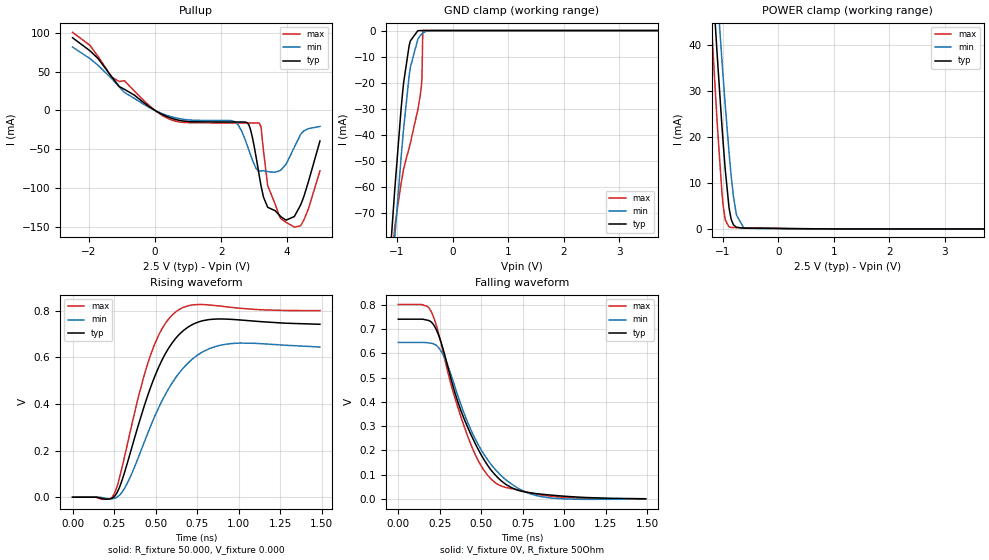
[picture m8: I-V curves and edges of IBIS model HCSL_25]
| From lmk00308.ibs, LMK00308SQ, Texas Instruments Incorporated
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|   Model HCSL_25
[Model]   HCSL_25
Model_type   Open_source
Polarity   Non-Inverting
Rref =   50.0000
Vref =   1.25
Vmeas =   1.25
|   typ   min   max
C_comp   1.5032pF   1.4574pF   1.5495pF
|Output in low   Nom   Weak   Strong
|C_Comp   1.5032pF   1.4574pF   1.5495pF
|Output in High   Nom   Strong   Weak
|C_Comp   1.0889pF   1.0724pF   1.10585pF
[Voltage Range]   2.5   2.375   2.625
[Temperature Range]   45   125   -40
[Pullup Reference]   2.5   2.375   2.625
[Pulldown Reference]   0   0   0
[Power Clamp Reference]   2.5   2.375   2.625
[GND Clamp Reference]   0   -0   0
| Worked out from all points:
|   slope of the pullup table from 0 to 0.375 V, typ, clamps not added: 46.2 ohm
|   GND clamp passes 1 mA (typ) near -0.66 V on its own axis
|   POWER clamp passes 1 mA (typ) near -0.81 V on its own axis
|   falling waveform, V_fixture 0V, R_fixture 50Ohm: 20-80 % time 248ps typ, 260ps min, 222ps max; typ from 0.74 V to 0.001 V
|   rising waveform, R_fixture 50.000, V_fixture 0.000: 20-80 % time 212ps typ, 251ps min, 177ps max; typ from 0 V to 0.742 V
[GND Clamp]
|   Voltage   I(typ)   I(min)   I(max)
-2.5V     -680.7mA   -652.3mA   -694.7mA
-1.135V   -89.97mA   -107.4mA   -101.7mA
-1.045V   -62.74mA   -81.12mA   -76.76mA
-1.038V   -60.54mA   -78.99mA   -75.08mA
-925mV    -30mA      -48.72mA   -58.7mA
-880mV    -20.04mA   -37.72mA   -53.1mA
-760mV    -4.036mA   -14.22mA   -43.38mA
-625mV    -70.9uA    -3.386mA   -30.51mA
-572.5mV  -12.45uA   -1.77mA    -23.42mA
-550mV    -6.1uA     -1.283mA   -18.23mA
-535mV    -3.82uA    -1.017mA   0A
4.992V    0A         0A         0A
[Pullup]
|   Voltage   I(typ)   I(min)   I(max)
-2.5V     93.46mA    81.56mA    100.4mA
-1.083V   30.64mA    30.07mA    37.19mA
320mV     -7.167mA   -5.716mA   -8.877mA
2.413V    -14.84mA   -14.44mA   -16.03mA
2.788V    -15.72mA   -44.64mA   -16.04mA
2.945V    -34.36mA   -63.37mA   -16.04mA
3.155V    -83.98mA   -78.14mA   -16.37mA
3.208V    -96.81mA   -77.83mA   -21.02mA
3.41V     -124.5mA   -78.7mA    -96.85mA
3.965V    -141.1mA   -69.18mA   -143.8mA
4.445V    -117.5mA   -28.91mA   -145.7mA
4.992V    -39.26mA   -20.58mA   -77.68mA
[POWER Clamp]
|   Voltage   I(typ)   I(min)   I(max)
-2.5V     367mA      361.7mA    377.1mA
-1.21V    59.59mA    72.33mA    46.61mA
-1.143V   46.29mA    59.65mA    32.09mA
-1.105V   39.1mA     52.81mA    24.38mA
-1.09V    36.27mA    50.11mA    21.4mA
-1.015V   22.74mA    37.01mA    8.205mA
-955mV    13.09mA    27.12mA    2.027mA
-880mV    4.226mA    15.88mA    429.9uA
-805mV    886.5uA    6.959mA    296.1uA
-752.5mV  360.6uA    3.052mA    282.5uA
-595mV    172.5uA    235uA      254.5uA
4.992V    0A         0A         0A
[Ramp]
R_load = 50
|   typ   min   max
dV/dt_r   0.445052/2.11691e-10   0.375444/2.50863e-10   0.480248/1.76981e-10
dV/dt_f   0.443208/2.481e-10   0.374851/2.59538e-10   0.479892/2.21825e-10
[Falling Waveform]
V_fixture = 0V
V_fixture_min = 0V
V_fixture_max = 0V
R_fixture = 50Ohm
C_fixture = 0F
|   Time   V(typ)   V(min)   V(max)
0s        739.9mV    644.3mV    800.4mV
195ps     730.4mV    641.3mV    775.8mV
275ps     605.4mV    587mV      589.8mV
350ps     418.7mV    443.9mV    396.7mV
420ps     292.4mV    312.8mV    255.4mV
495ps     187.5mV    207.8mV    141.6mV
580ps     102.3mV    125.1mV    69.72mV
685ps     45.97mV    60.45mV    42.44mV
855ps     20.63mV    10.73mV    17.56mV
1.49ns    1.24mV     0V         582.5uV
[Rising Waveform]
R_fixture = 50.000
V_fixture = 0.000
V_fixture_min = 0.000
V_fixture_max = 0.000
C_fixture = 0.000
|  time   V(typ)   V(min)   V(max)
0s        4.039uV    0V         11.67nV
245ps     -877.4uV   -5.681mV   6.978mV
280ps     37.94mV    7.194mV    75.48mV
325ps     134.3mV    53.69mV    210.6mV
465ps     461mV      295.9mV    599.3mV
540ps     589.9mV    415.1mV    723.7mV
625ps     684.5mV    516.6mV    796.8mV
735ps     745.1mV    600.4mV    825.6mV
880ps     764.5mV    650.3mV    820.6mV
1.49ns    741.8mV    644.3mV    800.4mV
